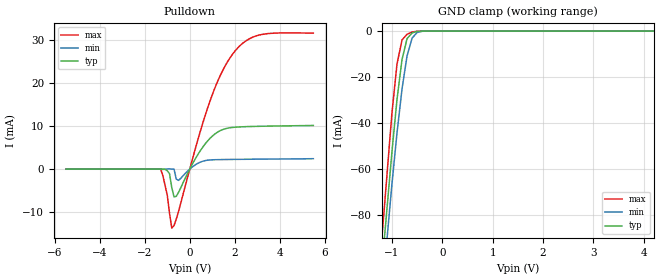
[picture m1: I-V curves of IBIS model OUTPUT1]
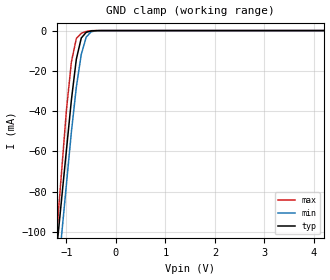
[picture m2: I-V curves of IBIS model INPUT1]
| IBIS file 4045sa.ibs
[IBIS ver]   3.0
[File name]   4045sa.ibs
[File Rev]   1.0
[Date]   Jul 05, 2005
[Source]   This file orginated at SEIKO EPSON QD Div.
[Copyright]   Copyright SEIKO EPSON Corp. 2005
|   Component 4045sa
[Component]   4045sa
[Manufacturer]   SEIKO EPSON
[Package]
| variable   typ   min   max
R_pkg   3.00m   NA   NA
L_pkg   3.70nH   NA   NA
C_pkg   0.70pF   NA   NA
[Pin]  signal_name   model_name   R_pin   L_pin   C_pin
|1   NC
2   CLK   INPUT1
3   FOUT   OUTPUT1
|4   NC
|5   TEST
6   VDD   POWER
| Models and submodels in the file (2): OUTPUT1 (Open_drain), INPUT1 (Input)
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|7   CE
|8   NC
|9   NC
|10   /INT
|11   GND
|12   DI
|13   DO
|14   NC
|   Model OUTPUT
[Model]   OUTPUT1
Model_type   Open_drain
Polarity   Non-Inverting
Enable   Active-High
Vmeas =   1.50V
C_comp   1.69pF   1.32pF   1.96pF
[Temperature Range]   25.00   85.00   -40.000
[Voltage Range]   3.0V   1.7V   5.5V
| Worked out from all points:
|   slope of the pulldown table from 0 to 0.45 V, typ, clamps not added: 110 ohm
|   GND clamp passes 1 mA (typ) near -0.61 V on its own axis
[Pulldown]
| voltage   I(typ)   I(min)   I(max)
-5.5V     0A         0A         0A
-1.3V     0A         0A         0A
-1V       -388uA     25uA       -6.092mA
-900mV    -1.083mA   53uA       -10.3mA
-800mV    -4.316mA   -17uA      -13.73mA
-700mV    -6.466mA   -23uA      -13.11mA
-600mV    -6.33mA    -2.33mA    -11.61mA
300mV     2.853mA    1.155mA    5.703mA
900mV     7.133mA    2.119mA    15.8mA
1.9V      9.676mA    2.242mA    26.66mA
3.1V      9.938mA    2.303mA    31.15mA
5.5V      10.13mA    2.41mA     31.58mA
[GND_clamp]
| voltage   I(typ)   I(min)   I(max)
-5.5V     -1.182A    -1.162A    -1.261A
-1.2V     -102.7mA   -115.2mA   -90.08mA
-1.1V     -77.56mA   -90.84mA   -62.86mA
-1V       -52.45mA   -66.5mA    -35.63mA
-900mV    -29.83mA   -44.41mA   -14.39mA
-800mV    -12.38mA   -25.18mA   -3.855mA
-700mV    -3.281mA   -10.8mA    -1.386mA
-600mV    -820uA     -3.055mA   -435uA
-500mV    -190uA     -606uA     -49uA
-300mV    0A         -7uA       0A
5.5V      0A         0A         0A
[Ramp]
| variable   typ   min   max
dV/dt_r 1.968/4.56n   0.874/16.96n   3.888/1.422n
dV/dt_f 1.968/4.56n   0.874/16.96n   3.888/1.422n
R_load = 500.00
| End [Model] OUTPUT
|   Model INPUT1
[Model]   INPUT1
Model_type   Input
Polarity   Non-Inverting
Vinl = 0.60V
Vinh = 2.40V
C_comp   0.80pF   0.60pF   1.00pF
[Temperature Range]   25.00   85.00   -40.00
[Voltage Range]   3.0V   1.7V   5.5V
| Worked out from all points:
|   GND clamp passes 1 mA (typ) near -0.60 V on its own axis
[GND_clamp]
| voltage   I(typ)   I(min)   I(max)
-5.5V     -1.179A    -1.245A    -1.443A
-1.2V     -109.2mA   -128.4mA   -102mA
-1.1V     -84.36mA   -102.4mA   -70.81mA
-1V       -59.47mA   -76.41mA   -39.62mA
-900mV    -34.59mA   -50.44mA   -15.66mA
-800mV    -14.24mA   -28.13mA   -3.931mA
-700mV    -3.678mA   -11.8mA    -1.351mA
-600mV    -868uA     -3.229mA   -419uA
-500mV    -202uA     -612uA     -46uA
-300mV    -1uA       -7uA       0A
5.5V      0A         0A         0A
